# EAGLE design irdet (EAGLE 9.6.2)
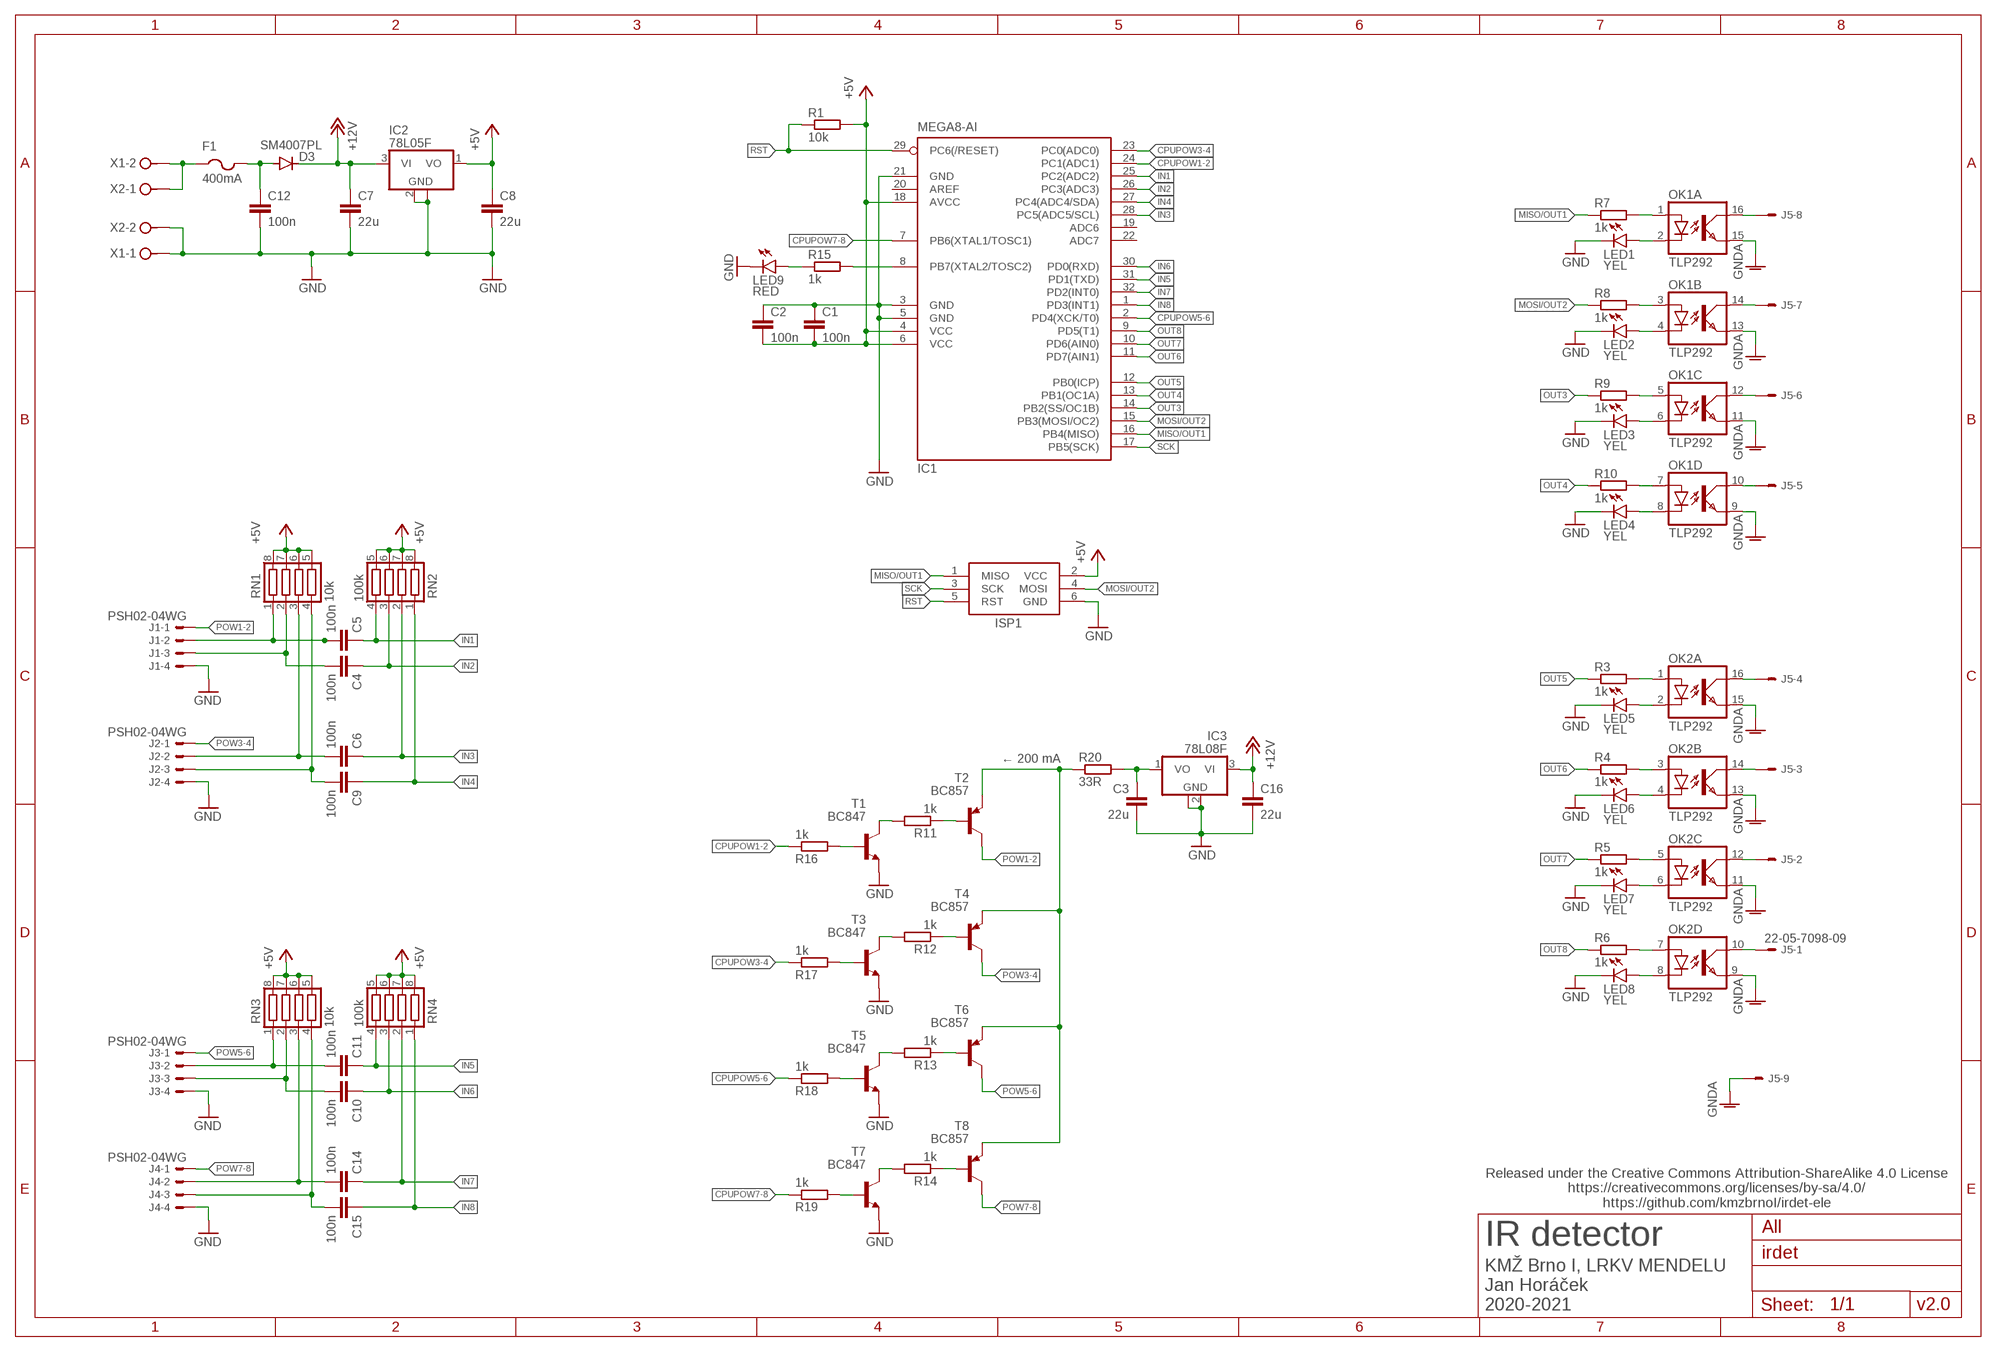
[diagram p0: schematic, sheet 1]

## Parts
C1  100n  C-EUC0805  [C0805]
C2  100n  C-EUC0805  [C0805]
C3  22u  C-EUC0805  [C0805]
C4  100n  C-EUC0805  [C0805]
C5  100n  C-EUC0805  [C0805]
C6  100n  C-EUC0805  [C0805]
C7  22u  C-EUC0805  [C0805]
C8  22u  C-EUC0805  [C0805]
C9  100n  C-EUC0805  [C0805]
C10  100n  C-EUC0805  [C0805]
C11  100n  C-EUC0805  [C0805]
C12  100n  C-EUC0805  [C0805]
C14  100n  C-EUC0805  [C0805]
C15  100n  C-EUC0805  [C0805]
C16  22u  C-EUC0805  [C0805]
D3  SM4007PL  CGRM4007-G  [SOD-123_MINI-SMA]
F1  400mA  PTCFUSE-0805  [R0805]
IC1  MEGA8-AI  [TQFP32-08]
IC2  78L05F  [SOT89]
IC3  78L08F  [SOT89]
ISP1  AVRISP-6  [AVRISP]
J1  PSH02-04WG  22-05-7048-04  [7395-04]
J2  PSH02-04WG  22-05-7048-04  [7395-04]
J3  PSH02-04WG  22-05-7048-04  [7395-04]
J4  PSH02-04WG  22-05-7048-04  [7395-04]
J5  22-05-7098-09  [7395-09]
LED1  YEL  LEDCHIPLED_0805  [CHIPLED_0805]
LED2  YEL  LEDCHIPLED_0805  [CHIPLED_0805]
LED3  YEL  LEDCHIPLED_0805  [CHIPLED_0805]
LED4  YEL  LEDCHIPLED_0805  [CHIPLED_0805]
LED5  YEL  LEDCHIPLED_0805  [CHIPLED_0805]
LED6  YEL  LEDCHIPLED_0805  [CHIPLED_0805]
LED7  YEL  LEDCHIPLED_0805  [CHIPLED_0805]
LED8  YEL  LEDCHIPLED_0805  [CHIPLED_0805]
LED9  RED  LEDCHIPLED_0805  [CHIPLED_0805]
OK1  TLP292  TLP283-4  [MINI-FLAT-16]
OK2  TLP292  TLP283-4  [MINI-FLAT-16]
R1  10k  R-EU_R0805  [R0805]
R3  1k  R-EU_R0805  [R0805]
R4  1k  R-EU_R0805  [R0805]
R5  1k  R-EU_R0805  [R0805]
R6  1k  R-EU_R0805  [R0805]
R7  1k  R-EU_R0805  [R0805]
R8  1k  R-EU_R0805  [R0805]
R9  1k  R-EU_R0805  [R0805]
R10  1k  R-EU_R0805  [R0805]
R11  1k  R-EU_R0805  [R0805]
R12  1k  R-EU_R0805  [R0805]
R13  1k  R-EU_R0805  [R0805]
R14  1k  R-EU_R0805  [R0805]
R15  1k  R-EU_R0805  [R0805]
R16  1k  R-EU_R0805  [R0805]
R17  1k  R-EU_R0805  [R0805]
R18  1k  R-EU_R0805  [R0805]
R19  1k  R-EU_R0805  [R0805]
R20  33R  R-EU_R2010  [R2010]
RN1  10k  CTS742C083  [CTS742C083]
RN2  100k  CTS742C083  [CTS742C083]
RN3  10k  CTS742C083  [CTS742C083]
RN4  100k  CTS742C083  [CTS742C083]
T1  BC847  BC808-NPN-SOT23-BEC  [SOT23-BEC]
T2  BC857  BC807-16-PNP-SOT23-BEC  [SOT23-BEC]
T3  BC847  BC808-NPN-SOT23-BEC  [SOT23-BEC]
T4  BC857  BC807-16-PNP-SOT23-BEC  [SOT23-BEC]
T5  BC847  BC808-NPN-SOT23-BEC  [SOT23-BEC]
T6  BC857  BC807-16-PNP-SOT23-BEC  [SOT23-BEC]
T7  BC847  BC808-NPN-SOT23-BEC  [SOT23-BEC]
T8  BC857  BC807-16-PNP-SOT23-BEC  [SOT23-BEC]
X1  MVE252-5-V  [MVE252-5-V]
X2  MVE252-5-V  [MVE252-5-V]

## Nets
+5V [power5V]: C1.2 C2.2 C8.1 IC1.4(VCC) IC1.6(VCC) IC1.18(AVCC) IC2.1(VO) ISP1.2(VCC) R1.2 RN1.5 RN1.6 RN1.7 RN1.8 RN2.5 RN2.6 RN2.7 RN2.8 RN3.5 RN3.6 RN3.7 RN3.8 RN4.5 RN4.6 RN4.7 RN4.8
+8V: C3.1 IC3.1(VO) R20.2
+12V: C7.1 C16.1 D3.C IC2.3(VI) IC3.3(VI)
+12VIN: F1.1 X1.2 X2.1
CPUPOW1-2: IC1.24(PC1(ADC1)) R16.1
CPUPOW3-4: IC1.23(PC0(ADC0)) R17.1
CPUPOW5-6: IC1.2(PD4(XCK/T0)) R18.1
CPUPOW7-8: IC1.7(PB6(XTAL1/TOSC1)) R19.1
GND: C1.1 C2.1 C3.2 C7.2 C8.2 C12.2 C16.2 IC1.3(GND) IC1.5(GND) IC1.21(GND) IC2.2(GND) IC2.2@1(GND) IC3.2(GND) IC3.2@1(GND) ISP1.6(GND) J1.4 J2.4 J3.4 J4.4 LED1.C LED2.C LED3.C LED4.C LED5.C LED6.C LED7.C LED8.C LED9.C T1.E T3.E T5.E T7.E X1.1 X2.2
GNDA: J5.9 OK1.9(D:EMIT) OK1.11(C:EMIT) OK1.13(B:EMIT) OK1.15(A:EMIT) OK2.9(D:EMIT) OK2.11(C:EMIT) OK2.13(B:EMIT) OK2.15(A:EMIT)
IN1: C5.1 IC1.25(PC2(ADC2)) RN2.4
IN2: C4.1 IC1.26(PC3(ADC3)) RN2.3
IN3: C6.1 IC1.28(PC5(ADC5/SCL)) RN2.2
IN4: C9.1 IC1.27(PC4(ADC4/SDA)) RN2.1
IN5: C11.1 IC1.31(PD1(TXD)) RN4.4
IN6: C10.1 IC1.30(PD0(RXD)) RN4.3
IN7: C14.1 IC1.32(PD2(INT0)) RN4.2
IN8: C15.1 IC1.1(PD3(INT1)) RN4.1
MISO/OUT1: IC1.16(PB4(MISO)) ISP1.1(MISO) R7.1
MOSI/OUT2: IC1.15(PB3(MOSI/OC2)) ISP1.4(MOSI) R8.1
N$1: C5.2 J1.2 RN1.1
N$2: C4.2 J1.3 RN1.2
N$3: C11.2 J3.2 RN3.1
N$4: C10.2 J3.3 RN3.2
N$5: C6.2 J2.2 RN1.3
N$6: C9.2 J2.3 RN1.4
N$7: C14.2 J4.2 RN3.3
N$8: C15.2 J4.3 RN3.4
N$9: LED5.A OK2.2(A:C)
N$10: OK2.1(A:A) R3.2
N$11: OK2.7(D:A) R6.2
N$12: OK2.5(C:A) R5.2
N$13: R11.1 T2.B
N$14: OK2.3(B:A) R4.2
N$15: LED6.A OK2.4(B:C)
N$16: LED7.A OK2.6(C:C)
N$17: LED8.A OK2.8(D:C)
N$18: LED1.A OK1.2(A:C)
N$19: OK1.1(A:A) R7.2
N$20: OK1.7(D:A) R10.2
N$21: OK1.5(C:A) R9.2
N$22: OK1.3(B:A) R8.2
N$23: LED2.A OK1.4(B:C)
N$24: LED3.A OK1.6(C:C)
N$25: LED4.A OK1.8(D:C)
N$26: J5.1 OK2.10(D:COL)
N$27: J5.2 OK2.12(C:COL)
N$28: J5.3 OK2.14(B:COL)
N$29: J5.4 OK2.16(A:COL)
N$30: J5.7 OK1.14(B:COL)
N$31: J5.8 OK1.16(A:COL)
N$32: J5.6 OK1.12(C:COL)
N$33: J5.5 OK1.10(D:COL)
N$34: IC1.8(PB7(XTAL2/TOSC2)) R15.2
N$35: R11.2 T1.C
N$36: R12.1 T4.B
N$37: R12.2 T3.C
N$38: R13.1 T6.B
N$39: R13.2 T5.C
N$40: R14.1 T8.B
N$41: R14.2 T7.C
N$42: R20.1 T2.E T4.E T6.E T8.E
N$47: LED9.A R15.1
N$48: R17.2 T3.B
N$49: R16.2 T1.B
N$50: R18.2 T5.B
N$51: R19.2 T7.B
N$58: C12.1 D3.A F1.2
OUT3: IC1.14(PB2(SS/OC1B)) R9.1
OUT4: IC1.13(PB1(OC1A)) R10.1
OUT5: IC1.12(PB0(ICP)) R3.1
OUT6: IC1.11(PD7(AIN1)) R4.1
OUT7: IC1.10(PD6(AIN0)) R5.1
OUT8: IC1.9(PD5(T1)) R6.1
POW1-2: J1.1 T2.C
POW3-4: J2.1 T4.C
POW5-6: J3.1 T6.C
POW7-8: J4.1 T8.C
RST: IC1.29(PC6(/RESET)) ISP1.5(RST) R1.1
SCK: IC1.17(PB5(SCK)) ISP1.3(SCK)
Unconnected: IC1.19(ADC6) IC1.20(AREF) IC1.22(ADC7)

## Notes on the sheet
- ← 200 mA
- Released under the Creative Commons Attribution-ShareAlike 4.0 License
  https://creativecommons.org/licenses/by-sa/4.0/
  https://github.com/kmzbrnoI/irdet-ele
- All
- IR detector
- KMŽ Brno I, LRKV MENDELU
  Jan Horáček
  2020-2021
- v2.0

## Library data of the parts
C1 C2 C4-C6 C9-C12 C14 C15 = rcl:C-EU: CAPACITOR, European symbol; LCSC_PART: C49478
C3 C7 C8 C16 = rcl:C-EU: CAPACITOR, European symbol; LCSC_PART: C45783
D3 = diode:CGRM400*-G: Molded plasitc,JEDEC SOD-123/Mini SMA; LCSC_PART: C64898
F1 = adafruit_edited:PTCFUSE: PTC fuses, resettable thermistors
IC1 = atmel:MEGA8: MICROCONTROLLER 8 Kbytes FLASH, 1 kbytes SRAM, 512 bytes EEPROM, USART, 6-channel 10 bit ADC, 2-channel 8 bit ADC Pin compatible with Atmega48, ATMega88, ATMega168 Source: avr.lbr; LCSC_PART: C14877; MPN: ATMEGA8-16AU; OC_FARNELL: 9171371; OC_NEWARK: 73M8863
IC2 = linear:78L*: POSITOIV-VOLTAGE REGULATORS Output up to 100 mA Source: Datasheet; LCSC_PART: C71136
IC3 = linear:78L*: POSITOIV-VOLTAGE REGULATORS Output up to 100 mA Source: Datasheet; LCSC_PART: C122846
ISP1 = adafruit:AVRISP: AVR ISP HEADER Standard 6 pin header for AVR programming
J1-J4 = con-molex:22-?-04: CONNECTOR wire to board 2.54 mm (.1 inch) pitch header; MF: MOLEX; OC_FARNELL: unknown; OC_NEWARK: unknown
J5 = con-molex:22-?-09: CONNECTOR wire to board 2.54 mm (.1 inch) pitch header; MF: MOLEX; OC_FARNELL: unknown; OC_NEWARK: unknown
LED1-LED9 = led:LED: LED
OK1 OK2 = optocoupler:TLP283-4: TOSHIBA PHOTOCOUPLER GaAs IRED & PHOTO-TRANSISTOR Source: http://www.semicon.toshiba.co.jp/td/en/Opto/Photocoupler/en_20050928_TLP283_datasheet.pdf; LCSC_PART: C95713; OC_FARNELL: unknown; OC_NEWARK: unknown
R1 = rcl:R-EU_: RESISTOR, European symbol; LCSC_PART: C17414
R3-R19 = rcl:R-EU_: RESISTOR, European symbol; LCSC_PART: C17513
R20 = rcl:R-EU_: RESISTOR, European symbol; SPICEPREFIX: R
RN1 RN3 = resistor-net:CTS742C083: Chip Resistor Array 4 Single Resistor Source: http://www.ctscorp.com/components/Datasheets/CTSChipArrayDs.pdf; LCSC_PART: C29718; OC_FARNELL: unknown; OC_NEWARK: unknown
RN2 RN4 = resistor-net:CTS742C083: Chip Resistor Array 4 Single Resistor Source: http://www.ctscorp.com/components/Datasheets/CTSChipArrayDs.pdf; LCSC_PART: C173315; OC_FARNELL: unknown; OC_NEWARK: unknown
T1 T3 T5 T7 = transistor:*-NPN-: NPN Transistror BF959 corrected 2008.03.06
T2 T4 T6 T8 = transistor:*-PNP-: PNP Transistror
X1 X2 = con-malina:MVE252-5-V

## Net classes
0 default: width 0.305 mm
1 mounthole: clearance 1 mm to class 0, clearance 1 mm
3 power5V: width 0.406 mm
4 power12V: width 0.406 mm, clearance 0.5 mm to class 0, clearance 0.5 mm to class 1, clearance 0.5 mm to class 2, clearance 0.5 mm to class 3

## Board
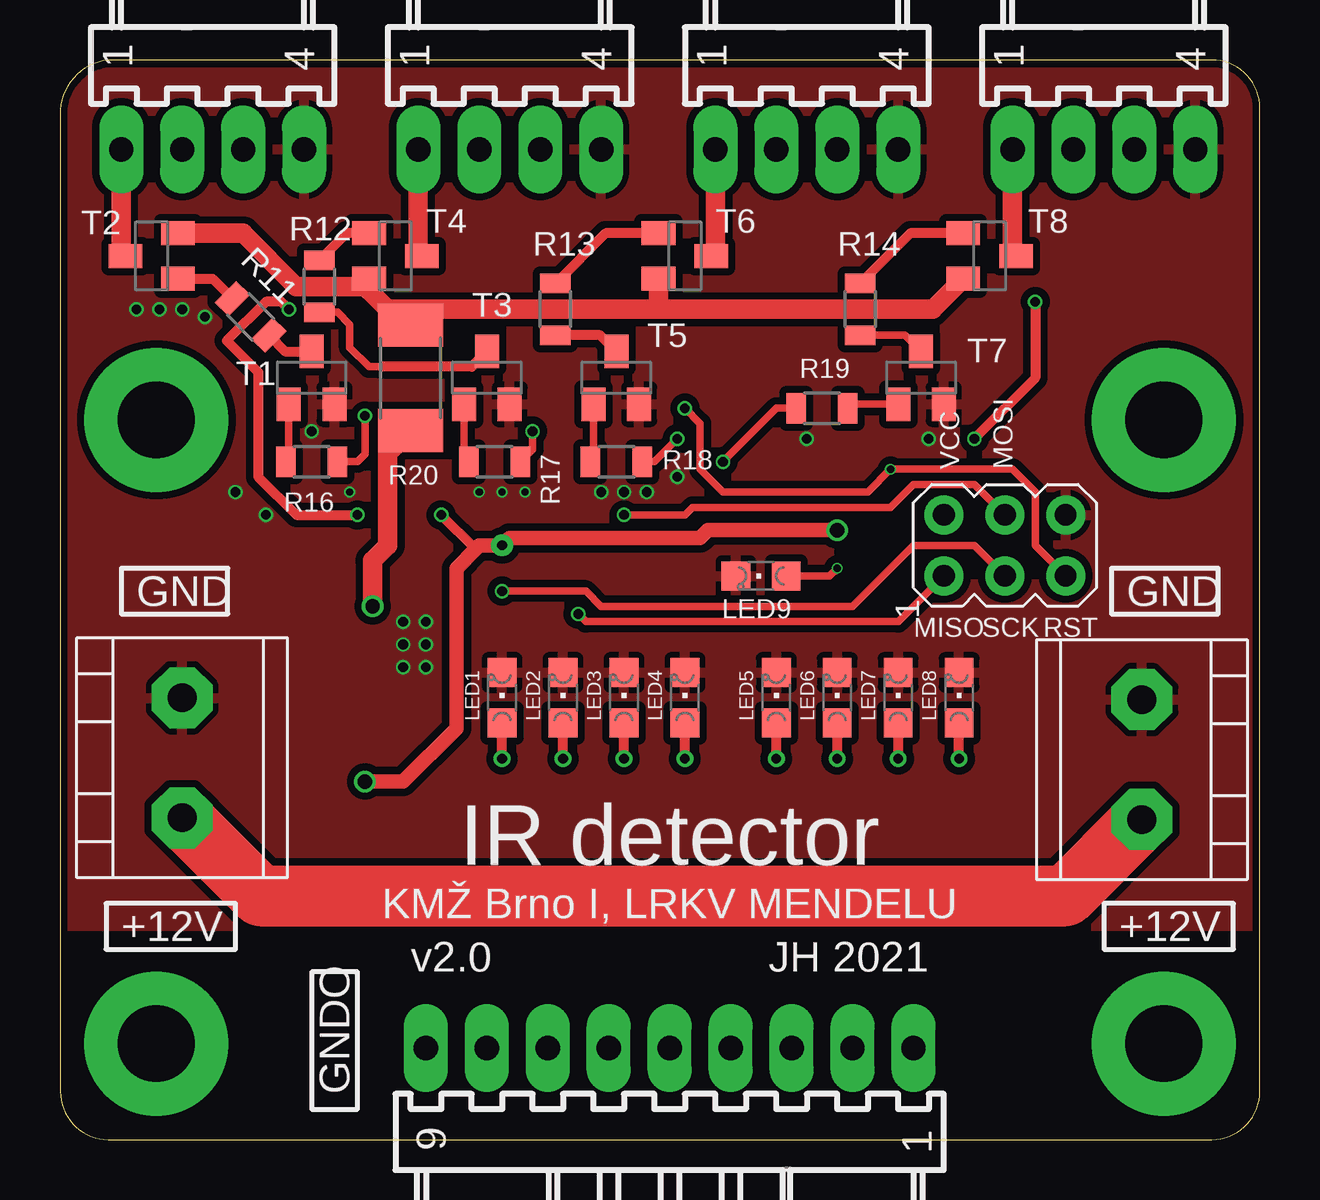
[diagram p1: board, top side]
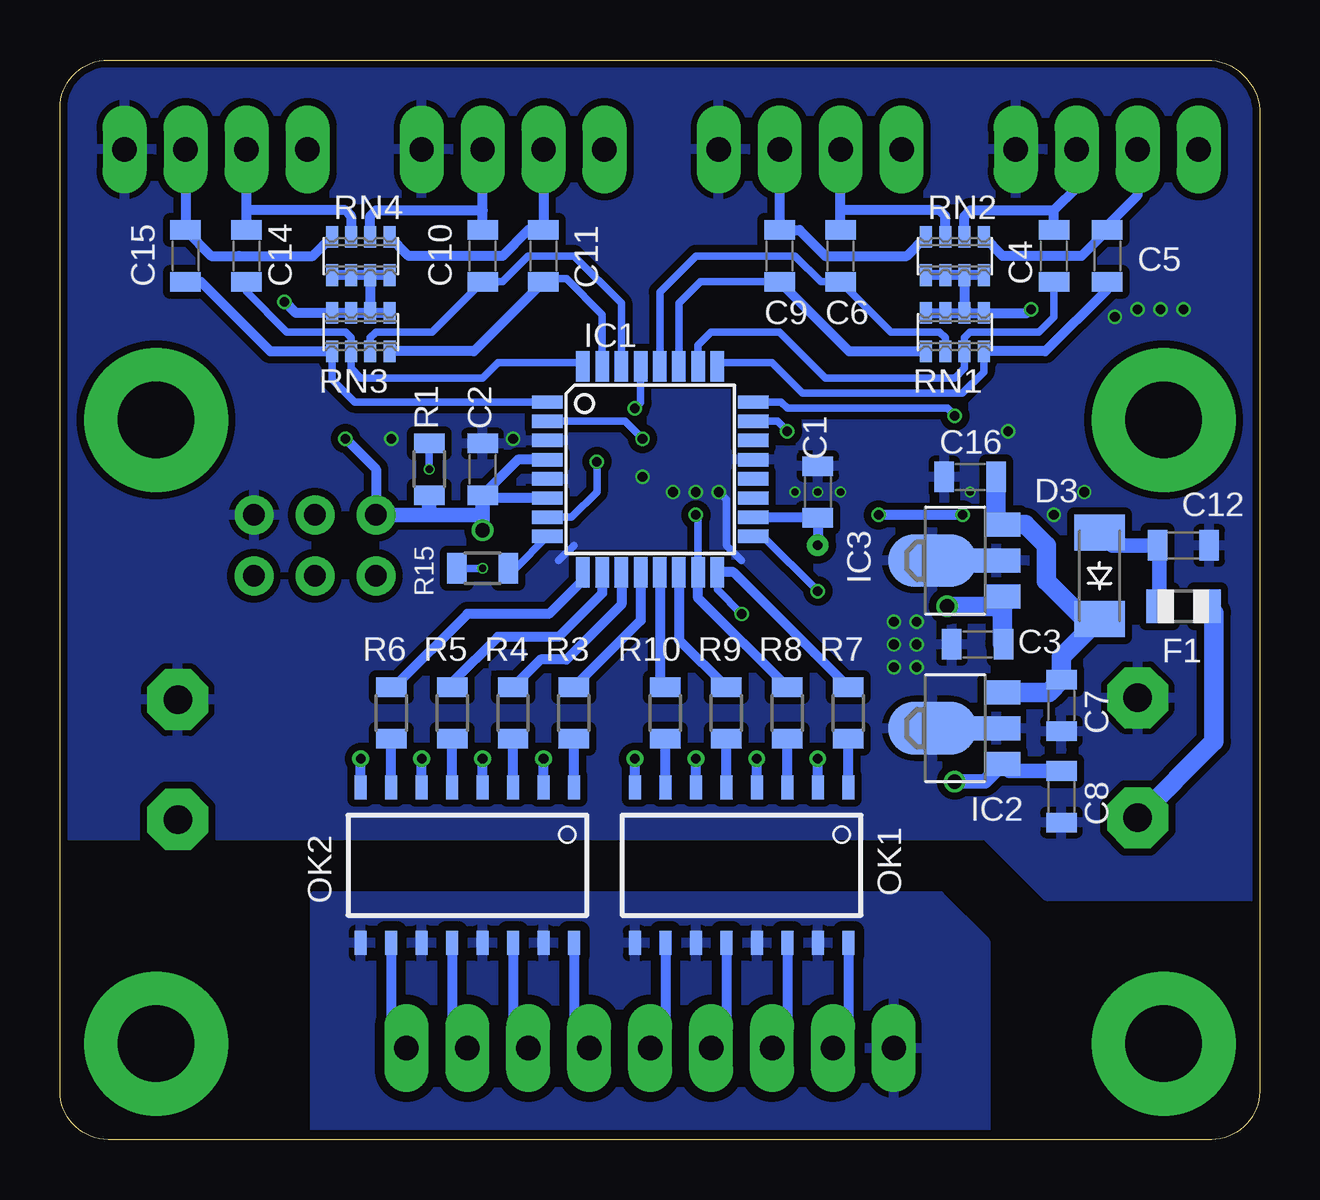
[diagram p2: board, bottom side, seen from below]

Size 50.01 x 45 mm. Coordinates in mm from the lower left corner, seen from the top.
Outline: 2.01,0 48.01,0 arc90 50.01,2 50.01,43 arc90 48.01,45 2.01,45 arc90 0.01,42.5 0.01,2 arc90 2.01,0
Copper layers (1*16): Top 0.035mm / dielectric 1.6mm / Bottom 0.035mm
Design rules "jlcpcb-2layers *": minimum track width 5mil, minimum drill 0.3mm, track to track 5mil, track to pad 5mil, pad to pad 5mil, via to via 5mil, smd to smd 5mil, copper to edge 0.2mm, drill to drill 6mil, minimum pad ring 10mil, minimum via ring 3mil, stop-mask expansion 4mil, vias tented up to drill 0.7mm, thermal gap 10mil

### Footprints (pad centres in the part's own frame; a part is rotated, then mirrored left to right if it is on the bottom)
C0805 = smd 0.813 x 1.27: 1 -1.077,0; 2 1.077,0
SOD-123_MINI-SMA = smd 1.5 x 2.1: A 1.8,0; C -1.8,0
R0805 = smd 1.1 x 1.4: 1 -1,0; 2 1,0
TQFP32-08 = smd 1.27 x 0.559: 1 -4.293,2.8; 2 -4.293,2; 3 -4.293,1.2; 4 -4.293,0.4; 5 -4.293,-0.4; 6 -4.293,-1.2; 7 -4.293,-2; 8 -4.293,-2.8; 17 4.293,-2.8; 18 4.293,-2; 19 4.293,-1.2; 20 4.293,-0.4; 21 4.293,0.4; 22 4.293,1.2; 23 4.293,2; 24 4.293,2.8 | smd 0.559 x 1.27: 9 -2.8,-4.293; 10 -2,-4.293; 11 -1.2,-4.293; 12 -0.4,-4.293; 13 0.4,-4.293; 14 1.2,-4.293; 15 2,-4.293; 16 2.8,-4.293; 25 2.8,4.293; 26 2,4.293; 27 1.2,4.293; 28 0.4,4.293; 29 -0.4,4.293; 30 -1.2,4.293; 31 -2,4.293; 32 -2.8,4.293
SOT89 = smd 1 x 1.5: 1 -1.499,-1.981; 3 1.499,-1.981 | smd 1 x 2: 2 0,-1.727 | smd 2.2 x 3.7: 2@1 0,0.94
AVRISP = drill 0.9 pad 1.626: 1 -1.27,2.54; 2 1.27,2.54; 3 -1.27,0; 4 1.27,0; 5 -1.27,-2.54; 6 1.27,-2.54
7395-04 = drill 1.016 long: 1 3.81,0; 2 1.27,0; 3 -1.27,0; 4 -3.81,0
7395-09 = drill 1.016 long: 1 10.16,0; 2 7.62,0; 3 5.08,0; 4 2.54,0; 5 0,0; 6 -2.54,0; 7 -5.08,0; 8 -7.62,0; 9 -10.16,0
CHIPLED_0805 = smd 1.2 x 1.2: A 0,-1.05; C 0,1.05
MINI-FLAT-16 = smd 1 x 0.5: 1 -3.24,4.445; 2 -3.24,3.175; 3 -3.24,1.905; 4 -3.24,0.635; 5 -3.24,-0.635; 6 -3.24,-1.905; 7 -3.24,-3.175; 8 -3.24,-4.445; 9 3.24,-4.445; 10 3.24,-3.175; 11 3.24,-1.905; 12 3.24,-0.635; 13 3.24,0.635; 14 3.24,1.905; 15 3.24,3.175; 16 3.24,4.445
R0805' = smd 0.813 x 1.27: 1 -1.077,0; 2 1.077,0
R2010 = smd 1.8 x 2.7: 1 -2.2,0; 2 2.2,0
CTS742C083 = smd 0.5 x 0.9: 1 -1.2,-0.8; 2 -0.4,-0.8; 3 0.4,-0.8; 4 1.2,-0.8; 5 1.2,0.8; 6 0.4,0.8; 7 -0.4,0.8; 8 -1.2,0.8
SOT23-BEC = smd 1 x 1.4: B -0.95,-1.1; C 0,1.1; E 0.95,-1.1
MVE252-5-V = drill 1.2 pad 2.54 octagon: 1 0,0; 2 5,0

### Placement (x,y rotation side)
C1  18.43,26.99 270 bottom
C2  32.4,27.94 270 bottom
C3  11.76,20.64 180 bottom
C4  8.59,36.83 90 bottom
C5  6.36,36.83 90 bottom
C6  17.48,36.83 90 bottom
C7  8.27,18.1 270 bottom
C8  8.27,14.29 270 bottom
C9  20.02,36.83 90 bottom
C10  32.4,36.83 90 bottom
C11  29.86,36.83 90 bottom
C12  3.19,24.77 0 bottom
C14  42.24,36.83 90 bottom
C15  44.78,36.83 90 bottom
C16  12.08,27.62 180 bottom
D3  6.68,23.5 90 bottom
F1  3.19,22.23 180 bottom
IC1  25.41,27.94 0 bottom
IC2  12.71,17.14 90 bottom
IC3  12.71,24.13 90 bottom
ISP1  39.38,24.77 90 top
J1  6.36,41.27 180 top
J2  18.75,41.27 180 top
J3  31.13,41.27 180 top
J4  43.51,41.27 180 top
J5  25.41,3.81 0 top
LED1  18.43,18.41 0 top
LED2  20.97,18.41 0 top
LED3  23.51,18.41 0 top
LED4  26.05,18.41 0 top
LED5  29.86,18.41 0 top
LED6  32.4,18.41 0 top
LED7  34.94,18.41 0 top
LED8  37.48,18.41 0 top
LED9  29.22,23.5 90 top
OK1  21.6,11.43 270 bottom
OK2  33.03,11.43 270 bottom
R1  10k  [R0805']  34.62,27.94 270 bottom
R3  1k  [R0805']  28.59,17.78 270 bottom
R4  1k  [R0805']  31.13,17.78 270 bottom
R5  1k  [R0805']  33.67,17.78 270 bottom
R6  1k  [R0805']  36.21,17.78 270 bottom
R7  1k  [R0805']  17.16,17.78 270 bottom
R8  1k  [R0805']  19.7,17.78 270 bottom
R9  1k  [R0805']  22.24,17.78 270 bottom
R10  1k  [R0805']  24.78,17.78 270 bottom
R11  1k  [R0805']  7.95,34.29 315 top
R12  1k  [R0805']  10.81,35.56 270 top
R13  1k  [R0805']  20.65,34.61 270 top
R14  1k  [R0805']  33.35,34.61 270 top
R15  1k  [R0805']  32.4,23.81 0 bottom
R16  1k  [R0805']  10.49,28.26 180 top
R17  1k  [R0805']  18.11,28.26 180 top
R18  1k  [R0805']  23.19,28.26 180 top
R19  1k  [R0805']  31.76,30.48 0 top
R20  14.62,31.75 270 top
RN1  12.71,36.83 180 bottom
RN2  12.71,33.66 0 bottom
RN3  37.48,36.83 180 bottom
RN4  37.48,33.66 0 bottom
T1  10.49,31.75 0 top
T2  3.82,36.83 90 top
T3  17.79,31.75 0 top
T4  13.98,36.83 270 top
T5  23.19,31.75 0 top
T6  26.05,36.83 270 top
T7  35.89,31.75 0 top
T8  38.75,36.83 270 top
X1  5.09,18.41 270 top
X2  45.1,13.34 90 top

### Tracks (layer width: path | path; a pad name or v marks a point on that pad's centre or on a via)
+5V  (via drill 0.4 pad 0.6, 0.4 pad 0.9, 0.6 pad 0.9)
  Top 0.406: v40.65,34.92 40.65,31.75 v38.11,29.21 | v9.54,34.61 9.22,34.92 8.59,34.92 6.95,33.29 8.27,31.98 8.27,27.62 9.86,26.04 v12.4,26.04 | 17.32,24.61 v15.89,26.04
  Top 0.61: v12.71,14.92 14.3,14.92 16.52,17.14 16.52,23.81 17.32,24.61 17.48,24.77 v18.43,24.77 18.75,25.08 26.68,25.08 27,25.4 v32.4,25.4
  Bottom 0.406: RN3.8 RN3.7 | RN3.7 RN3.6 RN3.5 | RN2.8 RN2.7 RN2.6 12.08,34.45 | 12.08,34.45 RN2.5 9.69,34.45 v9.54,34.61 | RN1.8 RN1.7 | RN1.7 RN1.6 RN1.5 | RN4.5 RN4.6 | RN4.6 RN4.7 RN4.8 40.18,34.45 v40.65,34.92 | RN1.7 12.31,34.69 12.08,34.45 | RN3.7 RN4.6 | IC1.18 18.46,25.94 C1.2 v18.43,24.77 | IC1.6 32.28,26.74 C2.2 30.92,28.34 IC1.4 | v38.11,29.21 36.84,27.94 ISP1.2 | v12.4,26.04 v15.89,26.04
  Bottom 0.61: C8.1 10.45,15.36 IC2.1 11.46,14.92 v12.71,14.92 | C2.2 32.4,26.04 | 32.4,26.04 v32.4,25.4 | ISP1.2 34.62,26.04 | 34.62,26.04 32.4,26.04 | R1.2 34.62,26.04
+8V  (via drill 0.6 pad 0.9)
  Top 0.813: R20.2 13.67,28.6 13.67,24.77 13.03,24.13 v13.03,22.23
  Bottom 0.813: C3.1 10.73,20.69 IC3.1 11.14,22.23 v13.03,22.23
+12V
  Bottom 0.813: IC2.3 8.8,18.64 C7.1 8.27,20.11 D3.C 7.32,21.7 8.9,23.28 8.9,24.77 9.77,25.63 IC3.3 11,25.9 C16.1
+12VIN
  Top 2.54: X1.2 8.35,10.16 41.92,10.16 X2.1
  Bottom 0.813: X1.2 1.92,16.59 1.92,21.95 F1.1
CPUPOW1-2  (via drill 0.4 pad 0.6)
  Top 0.305: v12.71,30.16 12.71,28.57 12.4,28.26 R16.1
  Bottom 0.305: IC1.24 19.96,30.74 19.7,30.48 13.03,30.48 v12.71,30.16
CPUPOW3-4  (via drill 0.4 pad 0.6)
  Top 0.305: v19.7,29.53 19.7,28.77 R17.1
  Bottom 0.305: IC1.23 20.11,29.94 v19.7,29.53
CPUPOW5-6  (via drill 0.4 pad 0.6)
  Top 0.305: v25.73,29.21 24.78,28.26 R18.1
  Bottom 0.305: IC1.2 26.46,29.94 v25.73,29.21
CPUPOW7-8  (via drill 0.4 pad 0.6)
  Top 0.305: v27.64,28.26 29.86,30.48 R19.1
  Bottom 0.305: IC1.7 28.68,25.94 27.64,26.99 v27.64,28.26
GND  (via drill 0.3, 0.4 pad 0.6)
  Bottom 0.305: 29.22,24.13 28.59,24.77 | 21.6,24.13 22.24,24.77 22.24,26.67 v22.56,26.99
  other vias: 17.48,26.99 18.43,26.99 19.38,26.99 14.3,19.68 15.25,19.68 14.3,20.64 15.25,20.64 15.25,21.59 14.3,21.59 23.51,26.99 25.73,27.62 24.46,26.99 31.13,29.21 36.21,29.21 10.49,29.53 12.08,26.99 7.32,26.99 6.05,34.29 5.09,34.61 4.14,34.61 3.19,34.61 8.59,26.04
  pour Bottom (isolate 0.305): -0.01,45.09 50.18,45.09 50.18,12.7 11.44,12.7 8.9,10.16 0,10.16
  pour Top (isolate 0.305): 0.01,45.09 50.18,45.09 50.18,8.89 0.01,8.89
GNDA
  pour Bottom (isolate 0.406): 11.44,0 39.38,0 39.38,10.16 13.35,10.16 11.44,8.26
IN1
  Bottom 0.305: RN2.4 11.51,32 12.4,31.11 19.06,31.11 20.33,32.38 22.46,32.38 IC1.25
  Bottom 0.406: C5.1 6.36,35.44 8.94,32.85 RN2.4
IN2
  Bottom 0.305: C4.1 8.59,34.29 9.22,33.66 12.08,33.66 12.31,33.42 RN2.3 12.31,32.15 12.71,31.75 18.11,31.75 20.02,33.66 22.87,33.66 23.41,33.12 IC1.26
IN3
  Bottom 0.305: RN2.2 13.11,33.42 13.35,33.66 15.38,33.66 C6.1 18.3,35.75 19.38,36.83 23.51,36.83 25.01,35.33 IC1.28
IN4
  Bottom 0.305: C9.1 23.32,35.75 24.21,34.85 IC1.27
  Bottom 0.406: C9.1 17.12,32.85 RN2.1
IN5
  Bottom 0.305: C11.1 29.73,35.88 28.91,35.88 27.41,34.38 IC1.31
  Bottom 0.406: C11.1 32.76,32.85 RN4.4
IN6
  Bottom 0.305: RN4.3 37.08,33.42 36.84,33.66 34.5,33.66 C10.1 31.57,35.75 30.49,36.83 28.59,36.83 26.61,34.85 IC1.30
IN7
  Bottom 0.305: C14.1 42.24,35.34 40.56,33.66 38.11,33.66 37.88,33.42 RN4.2 37.88,32.15 37.48,31.75 32.4,31.75 31.76,32.38 28.37,32.38 IC1.32
IN8
  Bottom 0.305: RN4.1 38.68,31.68 37.74,30.74 IC1.1
  Bottom 0.406: C15.1 44.15,35.75 41.25,32.85 RN4.1
MISO/OUT1  (via drill 0.4 pad 0.6)
  Top 0.305: ISP1.1 34.94,21.59 21.92,21.59 v21.6,21.91
  Bottom 0.305: v21.6,21.91 22.61,22.92 IC1.16
  Bottom 0.406: R7.1 21.95,23.65 IC1.16
MOSI/OUT2  (via drill 0.4 pad 0.6)
  Top 0.305: ISP1.4 38.11,27.3 35.57,27.3 34.62,26.35 26.37,26.35 26.05,26.04 v23.51,26.04
  Bottom 0.305: v23.51,26.04 23.41,25.94 IC1.15
  Bottom 0.406: R8.1 23.41,22.57 IC1.15
N$1
  Bottom 0.406: J1.2 5.09,39.37 6.36,38.1 C5.2 7.44,36.83 10.71,36.83 RN1.1
N$2
  Bottom 0.406: C4.2 8.59,38.73 | RN1.2 12.31,38.5 12.08,38.73 8.59,38.73 | J1.3 7.63,39.69 8.59,38.73
N$3
  Bottom 0.406: J3.2 C11.2 30.49,37.91 31.57,36.83 35.48,36.83 RN3.1
N$4
  Bottom 0.406: C10.2 32.4,38.73 | 32.4,38.73 J3.3 | RN3.2 37.08,38.5 36.84,38.73 32.4,38.73
N$5
  Bottom 0.406: C6.2 17.48,38.73 | 17.48,38.73 J2.2 | RN1.3 13.11,38.5 13.35,38.73 17.48,38.73
N$6
  Bottom 0.406: J2.3 C9.2 19.19,37.91 18.11,36.83 14.71,36.83 RN1.4
N$7
  Bottom 0.406: C14.2 42.24,38.73 | 42.24,38.73 J4.2 | RN3.3 37.88,38.5 38.11,38.73 42.24,38.73
N$8
  Bottom 0.406: J4.3 C15.2 43.7,36.83 42.56,36.83 39.48,36.83 RN3.4
N$9  (via drill 0.4 pad 0.7)
  Top 0.406: v29.86,15.88 LED5.A
  Bottom 0.406: OK2.2 v29.86,15.88
N$10
  Bottom 0.406: OK2.1 R3.2
N$11
  Bottom 0.406: OK2.7 R6.2
N$12
  Bottom 0.406: OK2.5 R5.2
N$13
  Top 0.406: T2.B 6.36,35.88 R11.1
N$14
  Bottom 0.406: OK2.3 R4.2
N$15  (via drill 0.4 pad 0.7)
  Top 0.406: v32.4,15.88 LED6.A
  Bottom 0.406: OK2.4 v32.4,15.88
N$16  (via drill 0.4 pad 0.7)
  Top 0.406: v34.94,15.88 LED7.A
  Bottom 0.406: OK2.6 v34.94,15.88
N$17  (via drill 0.4 pad 0.7)
  Top 0.406: v37.48,15.88 LED8.A
  Bottom 0.406: OK2.8 v37.48,15.88
N$18  (via drill 0.4 pad 0.7)
  Top 0.406: v18.43,15.88 LED1.A
  Bottom 0.406: OK1.2 v18.43,15.88
N$19
  Bottom 0.406: OK1.1 R7.2
N$20
  Bottom 0.406: OK1.7 R10.2
N$21
  Bottom 0.406: OK1.5 R9.2
N$22
  Bottom 0.406: OK1.3 R8.2
N$23  (via drill 0.4 pad 0.7)
  Top 0.406: v20.97,15.88 LED2.A
  Bottom 0.406: OK1.4 v20.97,15.88
N$24  (via drill 0.4 pad 0.7)
  Top 0.406: v23.51,15.88 LED3.A
  Bottom 0.406: OK1.6 v23.51,15.88
N$25  (via drill 0.4 pad 0.7)
  Top 0.406: v26.05,15.88 LED4.A
  Bottom 0.406: OK1.8 v26.05,15.88
N$26
  Bottom 0.406: OK2.10 36.21,4.45 J5.1
N$27
  Bottom 0.406: OK2.12 33.67,4.45 J5.2
N$28
  Bottom 0.406: OK2.14 31.13,4.45 J5.3
N$29
  Bottom 0.406: OK2.16 28.59,4.45 J5.4
N$30
  Bottom 0.406: OK1.14 19.7,4.45 J5.7
N$31
  Bottom 0.406: OK1.16 17.16,4.45 J5.8
N$32
  Bottom 0.406: OK1.12 22.24,4.45 J5.6
N$33
  Bottom 0.406: OK1.10 24.78,4.45 J5.5
N$34
  Bottom 0.305: IC1.8 31.03,23.81 R15.2
N$35
  Top 0.406: R11.2 9.39,32.85 T1.C
N$36
  Top 0.406: T4.B 11.95,37.78 R12.1
N$37
  Top 0.305: 13.39,32.22 12.88,32.22 12.08,33.02 12.08,33.97 11.57,34.48 11.13,34.48
  Top 0.406: T3.C 17.16,32.22 13.39,32.22 | 11.13,34.48 R12.2
N$38
  Top 0.406: T6.B 22.75,37.78 R13.1
N$39
  Top 0.406: T5.C 22.51,33.53 R13.2
N$40
  Top 0.406: T8.B 35.45,37.78 R14.1
N$41
  Top 0.305: R14.2 35.21,33.53 T7.C
N$42
  Top 0.813: 14.62,34.61 13.67,34.61 12.88,35.39 T4.E 12.57,35.56 9.85,35.56 7.64,37.78 T2.E | 14.62,34.61 25.1,34.61 | 25.1,34.61 36.38,34.61 T8.E | T6.E 24.95,34.76 25.1,34.61 | R20.1 14.62,34.61
N$43  (via drill 3.2 pad 6)
  other vias: 4.01,30
N$44  (via drill 3.2 pad 6)
  other vias: 46.01,30
N$45  (via drill 3.2 pad 6)
  other vias: 46.01,4
N$46  (via drill 3.2 pad 6)
  other vias: 4.01,4
N$47  (via drill 0.3)
  Top 0.305: v32.4,23.81 32.08,23.5 LED9.A
  Bottom 0.305: R15.1 v32.4,23.81
N$48
  Top 0.305: R17.2 16.84,28.45 T3.B
N$49
  Top 0.305: T1.B 9.54,28.38 R16.2
N$50
  Top 0.305: T5.B 22.24,28.38 R18.2
N$51
  Top 0.305: R19.2 33.01,30.65 T7.B
N$58
  Bottom 0.61: F1.2 4.19,24.69 C12.1 6.15,24.77 D3.A
OUT3
  Bottom 0.406: IC1.14 24.21,20.83 R9.1
OUT4
  Bottom 0.406: IC1.13 25.01,19.09 R10.1
OUT5
  Bottom 0.406: IC1.12 25.81,21.63 R3.1
OUT6
  Bottom 0.406: IC1.11 26.61,22.3 28.91,20 29.98,20 R4.1
OUT7
  Bottom 0.406: IC1.10 27.41,22.77 29.22,20.95 31.76,20.95 33.67,19.05 R5.1
OUT8
  Bottom 0.406: IC1.9 28.21,23.33 29.64,21.91 33.03,21.91 36.08,18.86 R6.1
POW1-2
  Top 0.813: T2.C 2.55,36.85 J1.1
POW3-4
  Top 0.813: T4.C 14.94,36.98 J2.1
POW5-6
  Top 0.813: T6.C 27.32,37 J3.1
POW7-8
  Top 0.813: T8.C 39.7,36.98 J4.1
RST  (via drill 0.3, 0.4 pad 0.6)
  Top 0.305: v26.05,30.48 26.68,29.84 26.68,27.94 27.64,26.99 33.67,26.99 v34.62,27.94 39.7,27.94 40.65,26.99 40.65,24.77 ISP1.5
  Bottom 0.305: R1.1 v34.62,27.94 | v26.05,30.48 25.81,30.71 IC1.29
SCK  (via drill 0.4 pad 0.6)
  Top 0.305: ISP1.3 38.11,24.77 35.57,24.77 33.03,22.23 22.56,22.23 21.92,22.86 v18.43,22.86
  Bottom 0.305: IC1.17 20.71,25.14 v18.43,22.86

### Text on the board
tNames: ⏚ | ⏚ | ⏚ | ⏚ | VCC | MOSI | ⏚ | GND | GND | MISO | SCK | RST | IR detector | KMŽ Brno I, LRKV MENDELU | +12V | +12V | v2.0 | JH 2021 | GNDO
